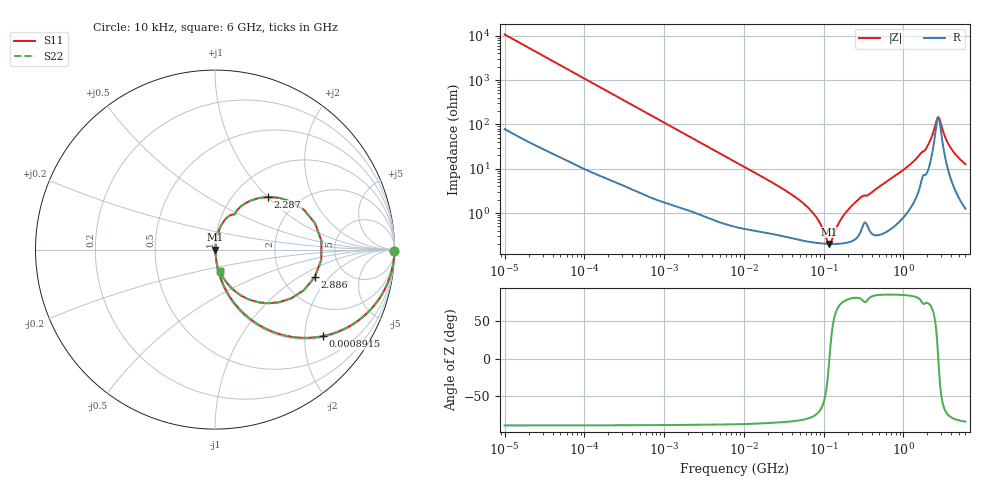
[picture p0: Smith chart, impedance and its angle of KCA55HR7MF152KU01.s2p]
!Murata Part Number: KCA55HR7MF152KU01
!These Parameters are Measured in Series Mode Connection
!Data Generated on Jan 08, 2026
!  o--ll--o
!Port1  Port2
!  o------o
!Operation Temp=25[degC], DC Bias Voltage=0[V]
!Freq. Start=10[kHz] Stop=6[GHz] 401[Steps]
# Hz S RI R 50
!Freq.(Hz) S11(Real) S11(Imag) S21(Real) S21(Imag) S12(Real) S12(Imag) S22(Real) S22(Imag)
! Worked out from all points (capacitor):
!   401 points, 10 kHz to 6 GHz, reference 50 ohm
!   read as one part in series: C = 1.48 nF near 10.69 kHz
!   lowest |Z| = 201 mohm at 118.5 MHz (marker M1)
!   series resonance near 118.3 MHz, so ESL is about 1.2 nH
!   S11 on the Smith chart (normalised r, x): 10 kHz: open; 891.5 kHz: 1.04, -2.47; 2.287 GHz: 1.42, +1.01; 2.886 GHz: 3.01, -1.39; 6 GHz: 1.03, -0.25
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10000  0.9998 -0.0093  0.000155 0.0093  0.000155 0.0093  0.9998 -0.0093
92862  0.992 -0.0847  0.008 0.0847  0.008 0.0847  0.992 -0.0847
351282  0.9039 -0.2888  0.0961 0.2888  0.0961 0.2888  0.9039 -0.2888
862344  0.6184 -0.4784  0.3816 0.4784  0.3816 0.4784  0.6184 -0.4784
891510  0.603 -0.4818  0.397 0.4818  0.397 0.4818  0.603 -0.4818
2499958  0.1711 -0.3656  0.8289 0.3656  0.8289 0.3656  0.1711 -0.3656
7745967  0.0252 -0.1407  0.9748 0.1407  0.9748 0.1407  0.0252 -0.1407
3.577363e7  0.00368 -0.0293  0.9963 0.0293  0.9963 0.0293  0.00368 -0.0293
7.193098e7  0.00229 -0.0103  0.9977 0.0103  0.9977 0.0103  0.00229 -0.0103
8.781895e7  0.00212 -0.00605  0.9979 0.00605  0.9979 0.00605  0.00212 -0.00605
1.184668e8  0.00201 3.49e-05  0.998 -3.49e-05  0.998 -3.49e-05  0.00201 3.49e-05
1.652154e8  0.00209 0.00693  0.9979 -0.00693  0.9979 -0.00693  0.00209 0.00693
2.228737e8  0.00248 0.014  0.9975 -0.014  0.9975 -0.014  0.00248 0.014
6.67969e8  0.00722 0.0556  0.9928 -0.0556  0.9928 -0.0556  0.00722 0.0556
1.534231e9  0.0592 0.1709  0.9408 -0.1709  0.9408 -0.1709  0.0592 0.1709
2.001953e9  0.1477 0.2437  0.8523 -0.2437  0.8523 -0.2437  0.1477 0.2437
2.286837e9  0.2969 0.2934  0.7031 -0.2934  0.7031 -0.2934  0.2969 0.2934
2.612262e9  0.5569 0.1475  0.4431 -0.1475  0.4431 -0.1475  0.5569 0.1475
2.886376e9  0.5552 -0.1545  0.4448 0.1545  0.4448 0.1545  0.5552 -0.1545
3.189254e9  0.3571 -0.2935  0.6429 0.2935  0.6429 0.2935  0.3571 -0.2935
3.766309e9  0.1483 -0.2574  0.8517 0.2574  0.8517 0.2574  0.1483 -0.2574
6e9  0.0276 -0.1216  0.9724 0.1216  0.9724 0.1216  0.0276 -0.1216
